| IBIS file stm32u595_599_5a5_5a9_ufbga132.ibs
[IBIS ver] 4.2
[File name] stm32u595_599_5a5_5a9_ufbga132.ibs
[File Rev] rev2.0
[Date]  11-09-2023
[Source] Data Created at STMicroelectronics
[Notes]  File originated from ELDO simulations.
[Disclaimer]  This information is for modeling purpose only and is
   not guaranteed. The information is subject to change without
   notice.
[Copyright] Copyright 2023 STMicroelectronics Inc.
|   Component stm32u595_599_5a5_5a9_ufbga132
[Component] stm32u595_599_5a5_5a9_ufbga132
[Manufacturer] STMicroelectronics
[Package]
| variable   typ   min   max
R_pkg  0  NA  NA
L_pkg  0  NA  NA
C_pkg  0  NA  NA
[Pin]   signal_name   model_name
A1  PE5  io8_100m_hslv_tamp_ft
A2  PE3  io8_100m_hslv_tamp_ft
A3  PE1  io8_100m_hslv_ft
A4  PB9  io8_100m_i2c_ft
A5  PB6  io8_100m_i2c_ft
A6  PG12  io8_100m_hslv_ft
A7  PD6  io8_166m_hslv_ft
A8  PD5  io8_100m_hslv_ft
A9  PD2  io8_100m_ft
A10  PC11  io8_100m_hslv_ft
A11  PA15  nc
A12  VDDUSB  power
B1  VBAT  power
B2  PE4  io8_100m_hslv_tamp_ft
B3  PE2  io8_100m_hslv_ft
B4  PG15  io8_100m_hslv_ft
B5  PH3-BOOT0  nc
B6  PB4  io8_100m_i2c_ft
B7  PG9  io8_100m_hslv_ft
B8  PD4  io8_100m_hslv_ft
B9  PD1  io8_100m_hslv_ft
B10  PC12  io8_166m_hslv_ft
B11  PC10  io8_100m_ft
B12  PA12  io8_100m_ft
C1  PC14-OSC32_IN  nc
C2  PE6  io8_100m_hslv_tamp_ft
C3  PC13  io8_100m_ft
C4  PE0  io8_100m_hslv_ft
C5  PB8  io8_100m_i2c_ft
C6  PB3  io8_100m_i2c_ft
C7  PG10  io8_100m_hslv_ft
C8  PD3  io8_166m_hslv_ft
C9  PD0  io8_100m_hslv_ft
C10  PA13  io8_100m_ft
C11  PA14  io8_100m_ft
C12  PA11  io8_100m_ft
D1  PC15-OSC32_OUT   nc
D2  PF0  io8_100m_hslv_ft
D3  PF3  io8_100m_hslv_ft
D4  VDD  power
D5  PB7  io8_spi_hslv_ft
D6  PB5  io8_166m_hslv_ft
D7  PD7  io8_100m_hslv_ft
D8  VDDIO2  power
D9  VDD  power
D10  PA9  io8_100m_usb_vbus_ft
D11  PA10  io8_100m_usb_id
D12  PA8  io8_166m_hslv_ft
E1  PF2  io8_100m_hslv_ft
E2  PF1  io8_100m_hslv_ft
E3  PF4  io8_spi_ft
E4  VSS  gnd
E9  VSS  gnd
E10  PC7  io8_100m_ft
E11  PC9  io8_100m_ft
E12  PC8  io8_100m_ft
F1  PH0-OSC_IN   nc
F2  PF5  io8_spi_ft
F3  PC2  io8_100m_hslv_ft
F4  PC3  io8_100m_hslv_ft
F6  VSS  gnd
F7  VDD  power
F9  PG6  io8_100m_hslv_ft
F10  PG7  io8_100m_hslv_ft
F11  PC6  io8_100m_ft
F12  PG8  io8_100m_i2c_ft
G1  PH1-OSC_OUT   nc
G2  NRST  nc
G3  PC1  io8_spi_hslv_ft
G4  PA1  io8_100m_hslv_tamp_ft
G6  VDD  power
G7  VSS  gnd
G9  PG4  io8_100m_hslv_ft
G10  PG2  io8_100m_hslv_ft
G11  PG3  io8_100m_hslv_ft
G12  PG5  io8_100m_hslv_ft
H1  VSSA_VREFM  nc
H2  PC0  io8_100m_hslv_ft
H3  OPAMP1_VINM  nc
H4  VSS  gnd
H9  VSS  gnd
H10  PD14  io8_100m_hslv_ft
H11  PD13  io8_100m_hslv_ft
H12  PD15  io8_100m_hslv_ft
J1  VREFP  nc
J2  PA0  io8_100m_hslv_tamp_ft
J3  PC5  io8_100m_tamp_ft
J4  VDD  power
J5  PF14  io8_100m_hslv_ft
J6  PE8  io8_100m_hslv_ft
J7  PE10  io8_166m_hslv_ft
J8  PE12  io8_100m_hslv_ft
J9  VDD  power
J10  PD9  io8_100m_hslv_ft
J11  PD11  io8_100m_hslv_ft
J12  PD12  io8_100m_hslv_ft
K1  VDDA  nc
K2  PA2  io8_100m_hslv_ft
K3  PA7  io8_100m_hslv_ft
K4  PB2  io8_100m_hslv_tamp_ft
K5  PF11  io8_166m_hslv_ft
K6  PG1  io8_100m_hslv_ft
K7  PE7  io8_100m_hslv_ft
K8  PE14  io8_100m_hslv_ft
K9  PB10  io8_spi_hslv_ft
K10  PB13  io8_100m_i2c_ft
K11  PB14  io8_100m_i2c_ft
K12  PB15  nc
L1  PA3  io8_166m_hslv_ft
L2  PA6  io8_100m_hslv_ft
L3  PA4  io8_100m_hslv_ft
L4  PB1  io8_100m_hslv_ft
L5  PF12  io8_100m_hslv_ft
L6  PF15  io8_100m_hslv_ft
L7  PE11  io8_100m_hslv_ft
L8  PE15  io8_100m_hslv_ft
L9  PB11  io8_100m_hslv_ft
L10  VCAP  nc
L11  PB12  io8_166m_hslv_ft
L12  PD8  io8_100m_hslv_ft
M1  PA5  io8_100m_ft
M2  OPAMP2_VINM  nc
M3  PC4  io8_100m_hslv_ft
M4  PB0  io8_100m_hslv_ft
M5  PF13  io8_100m_hslv_ft
M6  PG0  io8_100m_hslv_ft
M7  PE9  io8_166m_hslv_ft
M8  PE13  io8_100m_hslv_ft
M9  PG14  io8_100m_hslv_ft
M10  PG13  io8_100m_hslv_ft
M11  PG11  io8_100m_hslv_ft
M12  PD10  io8_100m_hslv_ft
[Package Model]   481-ufbga-7x7-132-ldo-220909
[Pin Mapping]   pulldown_ref   pullup_ref   | Comment
A1  gndio  vddiom
A2  gndio  vddiom
A3  gndio  vddiom
A4  gndio  vddiom
A5  gndio  vddiom
A6  gndio  vddiom  | Depending on IO usage
| A6  gndio  vddio2  | Depending on IO usage
A7  gndio  vddiom
A8  gndio  vddiom
A9  gndio  vddiom
A10  gndio  vddiom
A11  nc  nc
A12  nc  vddusb
B1  nc  vsw
B2  gndio  vddiom
B3  gndio  vddiom
B4  gndio  vddiom  | Depending on IO usage
| B4  gndio  vddio2  | Depending on IO usage
B5  nc  nc
B6  gndio  vddiom
B7  gndio  vddiom  | Depending on IO usage
| B7  gndio  vddio2  | Depending on IO usage
B8  gndio  vddiom
B9  gndio  vddiom
B10  gndio  vddiom
B11  gndio  vddiom
B12  gndio  vddiom  | Depending on IO usage
| B12  gndio  vddusb  | Depending on IO usage
C1  nc  nc
C2  gndio  vddiom
C3  gndio  vddiom  | Depending on IO usage
| C3  gndio  vsw  | Depending on IO usage
C4  gndio  vddiom
C5  gndio  vddiom
C6  gndio  vddiom
C7  gndio  vddiom  | Depending on IO usage
| C7  gndio  vddio2  | Depending on IO usage
C8  gndio  vddiom
C9  gndio  vddiom
C10  gndio  vddiom  | Depending on IO usage
| C10  gndio  vddusb  | Depending on IO usage
C11  gndio  vddiom
C12  gndio  vddiom  | Depending on IO usage
| C12  gndio  vddusb  | Depending on IO usage
D1  nc  nc
D2  gndio  vddiom
D3  gndio  vddiom
D4  nc  vddiom
D5  gndio  vddiom
D6  gndio  vddiom
D7  gndio  vddiom
D8  nc  vddio2
D9  nc  vddiom
D10  gndio  vddiom  | Depending on IO usage
| D10  gndio  vddusb  | Depending on IO usage
D11  gndio  vddiom  | Depending on IO usage
| D11  gndio  vddusb  | Depending on IO usage
D12  gndio  vddiom
E1  gndio  vddiom
E2  gndio  vddiom
E3  gndio  vddiom
E4  gndio  nc
E9  gndio  nc
E10  gndio  vddiom
E11  gndio  vddiom
E12  gndio  vddiom
F1  nc  nc
F2  gndio  vddiom
F3  gndio  vddiom
F4  gndio  vddiom
F6  gndio  nc
F7  nc  vddiom
F9  gndio  vddiom  | Depending on IO usage
| F9  gndio  vddio2  | Depending on IO usage
F10  gndio  vddiom  | Depending on IO usage
| F10  gndio  vddio2  | Depending on IO usage
F11  gndio  vddiom
F12  gndio  vddiom  | Depending on IO usage
| F12  gndio  vddio2  | Depending on IO usage
G1  nc  nc
G2  nc  nc
G3  gndio  vddiom
G4  gndio  vddiom
G6  nc  vddiom
G7  gndio  nc
G9  gndio  vddiom  | Depending on IO usage
| G9  gndio  vddio2  | Depending on IO usage
G10  gndio  vddiom  | Depending on IO usage
| G10  gndio  vddio2  | Depending on IO usage
G11  gndio  vddiom  | Depending on IO usage
| G11  gndio  vddio2  | Depending on IO usage
G12  gndio  vddiom  | Depending on IO usage
| G12  gndio  vddio2  | Depending on IO usage
H1  nc  nc
H2  gndio  vddiom
H3  nc  nc
H4  gndio  nc
H9  gndio  nc
H10  gndio  vddiom
H11  gndio  vddiom
H12  gndio  vddiom
J1  nc  nc
J2  gndio  vddiom
J3  gndio  vddiom
J4  nc  vddiom
J5  gndio  vddiom
J6  gndio  vddiom
J7  gndio  vddiom
J8  gndio  vddiom
J9  nc  vddiom
J10  gndio  vddiom
J11  gndio  vddiom
J12  gndio  vddiom
K1  nc  nc
K2  gndio  vddiom
K3  gndio  vddiom
K4  gndio  vddiom
K5  gndio  vddiom
K6  gndio  vddiom
K7  gndio  vddiom
K8  gndio  vddiom
K9  gndio  vddiom
K10  gndio  vddiom
K11  gndio  vddiom
K12  nc  nc
L1  gndio  vddiom
L2  gndio  vddiom
L3  gndio  vddiom
L4  gndio  vddiom
L5  gndio  vddiom
L6  gndio  vddiom
L7  gndio  vddiom
L8  gndio  vddiom
L9  gndio  vddiom
L10  nc  nc
L11  gndio  vddiom
L12  gndio  vddiom
M1  gndio  vddiom
M2  nc  nc
M3  gndio  vddiom
M4  gndio  vddiom
M5  gndio  vddiom
M6  gndio  vddiom
M7  gndio  vddiom
M8  gndio  vddiom
M9  gndio  vddiom  | Depending on IO usage
| M9  gndio  vddio2  | Depending on IO usage
M10  gndio  vddiom  | Depending on IO usage
| M10  gndio  vddio2  | Depending on IO usage
M11  gndio  vddiom  | Depending on IO usage
| M11  gndio  vddio2  | Depending on IO usage
M12  gndio  vddiom
[Model Selector] io8_100m_ft
io8_100m_ft_hs_1v2  "IO8_FT 100MHz high speed @ 1.2V"
io8_100m_ft_fs_1v2  "IO8_FT 100MHz fast speed @ 1.2V"
io8_100m_ft_fs_pd_1v2  "IO8_FT 100MHz fast speed @ 1.2V pulldown"
io8_100m_ft_ms_1v2  "IO8_FT 100MHz med speed @ 1.2V"
io8_100m_ft_ms_pd_1v2  "IO8_FT 100MHz med speed @ 1.2V pulldown"
io8_100m_ft_ls_1v2  "IO8_FT 100MHz low speed @ 1.2V"
io8_100m_ft_ls_pd_1v2  "IO8_FT 100MHz low speed @ 1.2V pulldown"
io8_100m_ft_hs_1v8  "IO8_FT 100MHz high speed @ 1.8V"
io8_100m_ft_hs_pd_1v8  "IO8_FT 100MHz high speed @ 1.8V pulldown"
io8_100m_ft_fs_1v8  "IO8_FT 100MHz fast speed @ 1.8V"
io8_100m_ft_fs_pd_1v8  "IO8_FT 100MHz fast speed @ 1.8V pulldown"
io8_100m_ft_ms_1v8  "IO8_FT 100MHz med speed @ 1.8V"
io8_100m_ft_ms_pd_1v8  "IO8_FT 100MHz med speed @ 1.8V pulldown"
io8_100m_ft_ls_1v8  "IO8_FT 100MHz low speed @ 1.8V"
io8_100m_ft_ls_pd_1v8  "IO8_FT 100MHz low speed @ 1.8V pulldown"
io8_100m_ft_hs_3v3  "IO8_FT 100MHz high speed @ 3.3V"
io8_100m_ft_hs_pd_3v3  "IO8_FT 100MHz high speed @ 3.3V pulldown"
io8_100m_ft_fs_3v3  "IO8_FT 100MHz fast speed @ 3.3V"
io8_100m_ft_fs_pd_3v3  "IO8_FT 100MHz fast speed @ 3.3V pulldown"
io8_100m_ft_ms_3v3  "IO8_FT 100MHz med speed @ 3.3V"
io8_100m_ft_ms_pd_3v3  "IO8_FT 100MHz med speed @ 3.3V pulldown"
io8_100m_ft_ls_3v3  "IO8_FT 100MHz low speed @ 3.3V"
io8_100m_ft_ls_pd_3v3  "IO8_FT 100MHz low speed @ 3.3V pulldown"
[Model Selector] io8_100m_hslv_ft
io8_100m_ft_hs_1v2  "IO8_FT 100MHz high speed @ 1.2V"
io8_100m_ft_hs_pu_1v2  "IO8_FT 100MHz high speed @ 1.2V pullup"
io8_100m_ft_hs_pd_1v2  "IO8_FT 100MHz high speed @ 1.2V pulldown"
io8_100m_ft_fs_1v2  "IO8_FT 100MHz fast speed @ 1.2V"
io8_100m_ft_fs_pu_1v2  "IO8_FT 100MHz fast speed @ 1.2V pullup"
io8_100m_ft_fs_pd_1v2  "IO8_FT 100MHz fast speed @ 1.2V pulldown"
io8_100m_ft_ms_1v2  "IO8_FT 100MHz med speed @ 1.2V"
io8_100m_ft_ms_pu_1v2  "IO8_FT 100MHz med speed @ 1.2V pullup"
io8_100m_ft_ms_pd_1v2  "IO8_FT 100MHz med speed @ 1.2V pulldown"
io8_100m_ft_ls_1v2  "IO8_FT 100MHz low speed @ 1.2V"
io8_100m_ft_ls_pu_1v2  "IO8_FT 100MHz low speed @ 1.2V pullup"
io8_100m_ft_ls_pd_1v2  "IO8_FT 100MHz low speed @ 1.2V pulldown"
io8_100m_ft_hs_1v8  "IO8_FT 100MHz high speed @ 1.8V"
io8_100m_ft_hs_pu_1v8  "IO8_FT 100MHz high speed @ 1.8V pullup"
io8_100m_ft_hs_pd_1v8  "IO8_FT 100MHz high speed @ 1.8V pulldown"
io8_100m_ft_fs_1v8  "IO8_FT 100MHz fast speed @ 1.8V"
io8_100m_ft_fs_pu_1v8  "IO8_FT 100MHz fast speed @ 1.8V pullup"
io8_100m_ft_fs_pd_1v8  "IO8_FT 100MHz fast speed @ 1.8V pulldown"
io8_100m_ft_ms_1v8  "IO8_FT 100MHz med speed @ 1.8V"
io8_100m_ft_ms_pu_1v8  "IO8_FT 100MHz med speed @ 1.8V pullup"
io8_100m_ft_ms_pd_1v8  "IO8_FT 100MHz med speed @ 1.8V pulldown"
io8_100m_ft_ls_1v8  "IO8_FT 100MHz low speed @ 1.8V"
io8_100m_ft_ls_pu_1v8  "IO8_FT 100MHz low speed @ 1.8V pullup"
io8_100m_ft_ls_pd_1v8  "IO8_FT 100MHz low speed @ 1.8V pulldown"
io8_100m_ft_hs_3v3  "IO8_FT 100MHz high speed @ 3.3V"
io8_100m_ft_hs_pu_3v3  "IO8_FT 100MHz high speed @ 3.3V pullup"
io8_100m_ft_hs_pd_3v3  "IO8_FT 100MHz high speed @ 3.3V pulldown"
io8_100m_ft_fs_3v3  "IO8_FT 100MHz fast speed @ 3.3V"
io8_100m_ft_fs_pu_3v3  "IO8_FT 100MHz fast speed @ 3.3V pullup"
io8_100m_ft_fs_pd_3v3  "IO8_FT 100MHz fast speed @ 3.3V pulldown"
io8_100m_ft_ms_3v3  "IO8_FT 100MHz med speed @ 3.3V"
io8_100m_ft_ms_pu_3v3  "IO8_FT 100MHz med speed @ 3.3V pullup"
io8_100m_ft_ms_pd_3v3  "IO8_FT 100MHz med speed @ 3.3V pulldown"
io8_100m_ft_ls_3v3  "IO8_FT 100MHz low speed @ 3.3V"
io8_100m_ft_ls_pu_3v3  "IO8_FT 100MHz low speed @ 3.3V pullup"
io8_100m_ft_ls_pd_3v3  "IO8_FT 100MHz low speed @ 3.3V pulldown"
io8_100m_hslv_ft_hs_1v2  "IO8_FT 100MHz HSLV high speed @ 1.2V"
io8_100m_hslv_ft_hs_pu_1v2  "IO8_FT 100MHz HSLV high speed @ 1.2V pullup"
io8_100m_hslv_ft_hs_pd_1v2  "IO8_FT 100MHz HSLV high speed @ 1.2V pulldown"
io8_100m_hslv_ft_fs_1v2  "IO8_FT 100MHz HSLV fast speed @ 1.2V"
io8_100m_hslv_ft_fs_pu_1v2  "IO8_FT 100MHz HSLV fast speed @ 1.2V pullup"
io8_100m_hslv_ft_fs_pd_1v2  "IO8_FT 100MHz HSLV fast speed @ 1.2V pulldown"
io8_100m_hslv_ft_ms_1v2  "IO8_FT 100MHz HSLV med speed @ 1.2V"
io8_100m_hslv_ft_ms_pu_1v2  "IO8_FT 100MHz HSLV med speed @ 1.2V pullup"
io8_100m_hslv_ft_ms_pd_1v2  "IO8_FT 100MHz HSLV med speed @ 1.2V pulldown"
io8_100m_hslv_ft_ls_1v2  "IO8_FT 100MHz HSLV low speed @ 1.2V"
io8_100m_hslv_ft_ls_pu_1v2  "IO8_FT 100MHz HSLV low speed @ 1.2V pullup"
io8_100m_hslv_ft_ls_pd_1v2  "IO8_FT 100MHz HSLV low speed @ 1.2V pulldown"
io8_100m_hslv_ft_hs_1v8  "IO8_FT 100MHz HSLV high speed @ 1.8V"
io8_100m_hslv_ft_hs_pu_1v8  "IO8_FT 100MHz HSLV high speed @ 1.8V pullup"
io8_100m_hslv_ft_hs_pd_1v8  "IO8_FT 100MHz HSLV high speed @ 1.8V pulldown"
io8_100m_hslv_ft_fs_1v8  "IO8_FT 100MHz HSLV fast speed @ 1.8V"
io8_100m_hslv_ft_fs_pu_1v8  "IO8_FT 100MHz HSLV fast speed @ 1.8V pullup"
io8_100m_hslv_ft_fs_pd_1v8  "IO8_FT 100MHz HSLV fast speed @ 1.8V pulldown"
io8_100m_hslv_ft_ms_1v8  "IO8_FT 100MHz HSLV med speed @ 1.8V"
io8_100m_hslv_ft_ms_pu_1v8  "IO8_FT 100MHz HSLV med speed @ 1.8V pullup"
io8_100m_hslv_ft_ms_pd_1v8  "IO8_FT 100MHz HSLV med speed @ 1.8V pulldown"
io8_100m_hslv_ft_ls_1v8  "IO8_FT 100MHz HSLV low speed @ 1.8V"
io8_100m_hslv_ft_ls_pu_1v8  "IO8_FT 100MHz HSLV low speed @ 1.8V pullup"
io8_100m_hslv_ft_ls_pd_1v8  "IO8_FT 100MHz HSLV low speed @ 1.8V pulldown"
io8_100m_hslv_ft_hs_2v5  "IO8_FT 100MHz HSLV high speed @ 2.5V"
io8_100m_hslv_ft_hs_pu_2v5  "IO8_FT 100MHz HSLV high speed @ 2.5V pullup"
io8_100m_hslv_ft_hs_pd_2v5  "IO8_FT 100MHz HSLV high speed @ 2.5V pulldown"
io8_100m_hslv_ft_fs_2v5  "IO8_FT 100MHz HSLV fast speed @ 2.5V"
io8_100m_hslv_ft_fs_pu_2v5  "IO8_FT 100MHz HSLV fast speed @ 2.5V pullup"
io8_100m_hslv_ft_fs_pd_2v5  "IO8_FT 100MHz HSLV fast speed @ 2.5V pulldown"
io8_100m_hslv_ft_ms_2v5  "IO8_FT 100MHz HSLV med speed @ 2.5V"
io8_100m_hslv_ft_ms_pu_2v5  "IO8_FT 100MHz HSLV med speed @ 2.5V pullup"
io8_100m_hslv_ft_ms_pd_2v5  "IO8_FT 100MHz HSLV med speed @ 2.5V pulldown"
io8_100m_hslv_ft_ls_2v5  "IO8_FT 100MHz HSLV low speed @ 2.5V"
io8_100m_hslv_ft_ls_pu_2v5  "IO8_FT 100MHz HSLV low speed @ 2.5V pullup"
io8_100m_hslv_ft_ls_pd_2v5  "IO8_FT 100MHz HSLV low speed @ 2.5V pulldown"
[Model Selector] io8_100m_hslv_tamp_ft
io8_100m_ft_hs_1v2  "IO8_FT 100MHz high speed @ 1.2V"
io8_100m_ft_hs_pu_1v2  "IO8_FT 100MHz high speed @ 1.2V pullup"
io8_100m_ft_hs_pd_1v2  "IO8_FT 100MHz high speed @ 1.2V pulldown"
io8_100m_ft_fs_1v2  "IO8_FT 100MHz fast speed @ 1.2V"
io8_100m_ft_fs_pu_1v2  "IO8_FT 100MHz fast speed @ 1.2V pullup"
io8_100m_ft_fs_pd_1v2  "IO8_FT 100MHz fast speed @ 1.2V pulldown"
io8_100m_ft_ms_1v2  "IO8_FT 100MHz med speed @ 1.2V"
io8_100m_ft_ms_pu_1v2  "IO8_FT 100MHz med speed @ 1.2V pullup"
io8_100m_ft_ms_pd_1v2  "IO8_FT 100MHz med speed @ 1.2V pulldown"
io8_100m_ft_ls_1v2  "IO8_FT 100MHz low speed @ 1.2V"
io8_100m_ft_ls_pu_1v2  "IO8_FT 100MHz low speed @ 1.2V pullup"
io8_100m_ft_ls_pd_1v2  "IO8_FT 100MHz low speed @ 1.2V pulldown"
io8_100m_ft_hs_1v8  "IO8_FT 100MHz high speed @ 1.8V"
io8_100m_ft_hs_pu_1v8  "IO8_FT 100MHz high speed @ 1.8V pullup"
io8_100m_ft_hs_pd_1v8  "IO8_FT 100MHz high speed @ 1.8V pulldown"
io8_100m_ft_fs_1v8  "IO8_FT 100MHz fast speed @ 1.8V"
io8_100m_ft_fs_pu_1v8  "IO8_FT 100MHz fast speed @ 1.8V pullup"
io8_100m_ft_fs_pd_1v8  "IO8_FT 100MHz fast speed @ 1.8V pulldown"
io8_100m_ft_ms_1v8  "IO8_FT 100MHz med speed @ 1.8V"
io8_100m_ft_ms_pu_1v8  "IO8_FT 100MHz med speed @ 1.8V pullup"
io8_100m_ft_ms_pd_1v8  "IO8_FT 100MHz med speed @ 1.8V pulldown"
io8_100m_ft_ls_1v8  "IO8_FT 100MHz low speed @ 1.8V"
io8_100m_ft_ls_pu_1v8  "IO8_FT 100MHz low speed @ 1.8V pullup"
io8_100m_ft_ls_pd_1v8  "IO8_FT 100MHz low speed @ 1.8V pulldown"
io8_100m_ft_hs_3v3  "IO8_FT 100MHz high speed @ 3.3V"
io8_100m_ft_hs_pu_3v3  "IO8_FT 100MHz high speed @ 3.3V pullup"
io8_100m_ft_hs_pd_3v3  "IO8_FT 100MHz high speed @ 3.3V pulldown"
io8_100m_ft_fs_3v3  "IO8_FT 100MHz fast speed @ 3.3V"
io8_100m_ft_fs_pu_3v3  "IO8_FT 100MHz fast speed @ 3.3V pullup"
io8_100m_ft_fs_pd_3v3  "IO8_FT 100MHz fast speed @ 3.3V pulldown"
io8_100m_ft_ms_3v3  "IO8_FT 100MHz med speed @ 3.3V"
io8_100m_ft_ms_pu_3v3  "IO8_FT 100MHz med speed @ 3.3V pullup"
io8_100m_ft_ms_pd_3v3  "IO8_FT 100MHz med speed @ 3.3V pulldown"
io8_100m_ft_ls_3v3  "IO8_FT 100MHz low speed @ 3.3V"
io8_100m_ft_ls_pu_3v3  "IO8_FT 100MHz low speed @ 3.3V pullup"
io8_100m_ft_ls_pd_3v3  "IO8_FT 100MHz low speed @ 3.3V pulldown"
io8_100m_hslv_ft_hs_1v2  "IO8_FT 100MHz HSLV high speed @ 1.2V"
io8_100m_hslv_ft_hs_pu_1v2  "IO8_FT 100MHz HSLV high speed @ 1.2V pullup"
io8_100m_hslv_ft_hs_pd_1v2  "IO8_FT 100MHz HSLV high speed @ 1.2V pulldown"
io8_100m_hslv_ft_fs_1v2  "IO8_FT 100MHz HSLV fast speed @ 1.2V"
io8_100m_hslv_ft_fs_pu_1v2  "IO8_FT 100MHz HSLV fast speed @ 1.2V pullup"
io8_100m_hslv_ft_fs_pd_1v2  "IO8_FT 100MHz HSLV fast speed @ 1.2V pulldown"
io8_100m_hslv_ft_ms_1v2  "IO8_FT 100MHz HSLV med speed @ 1.2V"
io8_100m_hslv_ft_ms_pu_1v2  "IO8_FT 100MHz HSLV med speed @ 1.2V pullup"
io8_100m_hslv_ft_ms_pd_1v2  "IO8_FT 100MHz HSLV med speed @ 1.2V pulldown"
io8_100m_hslv_ft_ls_1v2  "IO8_FT 100MHz HSLV low speed @ 1.2V"
io8_100m_hslv_ft_ls_pu_1v2  "IO8_FT 100MHz HSLV low speed @ 1.2V pullup"
io8_100m_hslv_ft_ls_pd_1v2  "IO8_FT 100MHz HSLV low speed @ 1.2V pulldown"
io8_100m_hslv_ft_hs_1v8  "IO8_FT 100MHz HSLV high speed @ 1.8V"
io8_100m_hslv_ft_hs_pu_1v8  "IO8_FT 100MHz HSLV high speed @ 1.8V pullup"
io8_100m_hslv_ft_hs_pd_1v8  "IO8_FT 100MHz HSLV high speed @ 1.8V pulldown"
io8_100m_hslv_ft_fs_1v8  "IO8_FT 100MHz HSLV fast speed @ 1.8V"
io8_100m_hslv_ft_fs_pu_1v8  "IO8_FT 100MHz HSLV fast speed @ 1.8V pullup"
io8_100m_hslv_ft_fs_pd_1v8  "IO8_FT 100MHz HSLV fast speed @ 1.8V pulldown"
io8_100m_hslv_ft_ms_1v8  "IO8_FT 100MHz HSLV med speed @ 1.8V"
io8_100m_hslv_ft_ms_pu_1v8  "IO8_FT 100MHz HSLV med speed @ 1.8V pullup"
io8_100m_hslv_ft_ms_pd_1v8  "IO8_FT 100MHz HSLV med speed @ 1.8V pulldown"
io8_100m_hslv_ft_ls_1v8  "IO8_FT 100MHz HSLV low speed @ 1.8V"
io8_100m_hslv_ft_ls_pu_1v8  "IO8_FT 100MHz HSLV low speed @ 1.8V pullup"
io8_100m_hslv_ft_ls_pd_1v8  "IO8_FT 100MHz HSLV low speed @ 1.8V pulldown"
io8_100m_hslv_ft_hs_2v5  "IO8_FT 100MHz HSLV high speed @ 2.5V"
io8_100m_hslv_ft_hs_pu_2v5  "IO8_FT 100MHz HSLV high speed @ 2.5V pullup"
io8_100m_hslv_ft_hs_pd_2v5  "IO8_FT 100MHz HSLV high speed @ 2.5V pulldown"
io8_100m_hslv_ft_fs_2v5  "IO8_FT 100MHz HSLV fast speed @ 2.5V"
io8_100m_hslv_ft_fs_pu_2v5  "IO8_FT 100MHz HSLV fast speed @ 2.5V pullup"
io8_100m_hslv_ft_fs_pd_2v5  "IO8_FT 100MHz HSLV fast speed @ 2.5V pulldown"
io8_100m_hslv_ft_ms_2v5  "IO8_FT 100MHz HSLV med speed @ 2.5V"
io8_100m_hslv_ft_ms_pu_2v5  "IO8_FT 100MHz HSLV med speed @ 2.5V pullup"
io8_100m_hslv_ft_ms_pd_2v5  "IO8_FT 100MHz HSLV med speed @ 2.5V pulldown"
io8_100m_hslv_ft_ls_2v5  "IO8_FT 100MHz HSLV low speed @ 2.5V"
io8_100m_hslv_ft_ls_pu_2v5  "IO8_FT 100MHz HSLV low speed @ 2.5V pullup"
io8_100m_hslv_ft_ls_pd_2v5  "IO8_FT 100MHz HSLV low speed @ 2.5V pulldown"
io8_ft_v33_hs_1v2  "IO8_FT_V33 high speed @ 1.2V"
io8_ft_v33_hs_pu_1v2  "IO8_FT_V33 high speed @ 1.2V pullup"
io8_ft_v33_hs_pd_1v2  "IO8_FT_V33 high speed @ 1.2V pulldown"
io8_ft_v33_fs_1v2  "IO8_FT_V33 fast speed @ 1.2V"
io8_ft_v33_fs_pu_1v2  "IO8_FT_V33 fast speed @ 1.2V pullup"
io8_ft_v33_fs_pd_1v2  "IO8_FT_V33 fast speed @ 1.2V pulldown"
io8_ft_v33_ms_1v2  "IO8_FT_V33 med speed @ 1.2V"
io8_ft_v33_ms_pu_1v2  "IO8_FT_V33 med speed @ 1.2V pullup"
io8_ft_v33_ms_pd_1v2  "IO8_FT_V33 med speed @ 1.2V pulldown"
io8_ft_v33_ls_1v2  "IO8_FT_V33 low speed @ 1.2V"
io8_ft_v33_ls_pu_1v2  "IO8_FT_V33 low speed @ 1.2V pullup"
io8_ft_v33_ls_pd_1v2  "IO8_FT_V33 low speed @ 1.2V pulldown"
io8_ft_v33_hs_1v8  "IO8_FT_V33 high speed @ 1.8V"
io8_ft_v33_hs_pu_1v8  "IO8_FT_V33 high speed @ 1.8V pullup"
io8_ft_v33_hs_pd_1v8  "IO8_FT_V33 high speed @ 1.8V pulldown"
io8_ft_v33_fs_1v8  "IO8_FT_V33 fast speed @ 1.8V"
io8_ft_v33_fs_pu_1v8  "IO8_FT_V33 fast speed @ 1.8V pullup"
io8_ft_v33_fs_pd_1v8  "IO8_FT_V33 fast speed @ 1.8V pulldown"
io8_ft_v33_ms_1v8  "IO8_FT_V33 med speed @ 1.8V"
io8_ft_v33_ms_pu_1v8  "IO8_FT_V33 med speed @ 1.8V pullup"
io8_ft_v33_ms_pd_1v8  "IO8_FT_V33 med speed @ 1.8V pulldown"
io8_ft_v33_ls_1v8  "IO8_FT_V33 low speed @ 1.8V"
io8_ft_v33_ls_pu_1v8  "IO8_FT_V33 low speed @ 1.8V pullup"
io8_ft_v33_ls_pd_1v8  "IO8_FT_V33 low speed @ 1.8V pulldown"
io8_ft_v33_hs_3v3  "IO8_FT_V33 high speed @ 3.3V"
io8_ft_v33_hs_pu_3v3  "IO8_FT_V33 high speed @ 3.3V pullup"
io8_ft_v33_hs_pd_3v3  "IO8_FT_V33 high speed @ 3.3V pulldown"
io8_ft_v33_fs_3v3  "IO8_FT_V33 fast speed @ 3.3V"
io8_ft_v33_fs_pu_3v3  "IO8_FT_V33 fast speed @ 3.3V pullup"
io8_ft_v33_fs_pd_3v3  "IO8_FT_V33 fast speed @ 3.3V pulldown"
io8_ft_v33_ms_3v3  "IO8_FT_V33 med speed @ 3.3V"
io8_ft_v33_ms_pu_3v3  "IO8_FT_V33 med speed @ 3.3V pullup"
io8_ft_v33_ms_pd_3v3  "IO8_FT_V33 med speed @ 3.3V pulldown"
io8_ft_v33_ls_3v3  "IO8_FT_V33 low speed @ 3.3V"
io8_ft_v33_ls_pu_3v3  "IO8_FT_V33 low speed @ 3.3V pullup"
io8_ft_v33_ls_pd_3v3  "IO8_FT_V33 low speed @ 3.3V pulldown"
[Model Selector] io8_100m_i2c_ft
io8_100m_ft_hs_1v2  "IO8_FT 100MHz high speed @ 1.2V"
io8_100m_ft_hs_pu_1v2  "IO8_FT 100MHz high speed @ 1.2V pullup"
io8_100m_ft_hs_pd_1v2  "IO8_FT 100MHz high speed @ 1.2V pulldown"
io8_100m_ft_fs_1v2  "IO8_FT 100MHz fast speed @ 1.2V"
io8_100m_ft_fs_pu_1v2  "IO8_FT 100MHz fast speed @ 1.2V pullup"
io8_100m_ft_fs_pd_1v2  "IO8_FT 100MHz fast speed @ 1.2V pulldown"
io8_100m_ft_ms_1v2  "IO8_FT 100MHz med speed @ 1.2V"
io8_100m_ft_ms_pu_1v2  "IO8_FT 100MHz med speed @ 1.2V pullup"
io8_100m_ft_ms_pd_1v2  "IO8_FT 100MHz med speed @ 1.2V pulldown"
io8_100m_ft_ls_1v2  "IO8_FT 100MHz low speed @ 1.2V"
io8_100m_ft_ls_pu_1v2  "IO8_FT 100MHz low speed @ 1.2V pullup"
io8_100m_ft_ls_pd_1v2  "IO8_FT 100MHz low speed @ 1.2V pulldown"
io8_100m_ft_hs_1v8  "IO8_FT 100MHz high speed @ 1.8V"
io8_100m_ft_hs_pu_1v8  "IO8_FT 100MHz high speed @ 1.8V pullup"
io8_100m_ft_hs_pd_1v8  "IO8_FT 100MHz high speed @ 1.8V pulldown"
io8_100m_ft_fs_1v8  "IO8_FT 100MHz fast speed @ 1.8V"
io8_100m_ft_fs_pu_1v8  "IO8_FT 100MHz fast speed @ 1.8V pullup"
io8_100m_ft_fs_pd_1v8  "IO8_FT 100MHz fast speed @ 1.8V pulldown"
io8_100m_ft_ms_1v8  "IO8_FT 100MHz med speed @ 1.8V"
io8_100m_ft_ms_pu_1v8  "IO8_FT 100MHz med speed @ 1.8V pullup"
io8_100m_ft_ms_pd_1v8  "IO8_FT 100MHz med speed @ 1.8V pulldown"
io8_100m_ft_ls_1v8  "IO8_FT 100MHz low speed @ 1.8V"
io8_100m_ft_ls_pu_1v8  "IO8_FT 100MHz low speed @ 1.8V pullup"
io8_100m_ft_ls_pd_1v8  "IO8_FT 100MHz low speed @ 1.8V pulldown"
io8_100m_ft_hs_3v3  "IO8_FT 100MHz high speed @ 3.3V"
io8_100m_ft_hs_pu_3v3  "IO8_FT 100MHz high speed @ 3.3V pullup"
io8_100m_ft_hs_pd_3v3  "IO8_FT 100MHz high speed @ 3.3V pulldown"
io8_100m_ft_fs_3v3  "IO8_FT 100MHz fast speed @ 3.3V"
io8_100m_ft_fs_pu_3v3  "IO8_FT 100MHz fast speed @ 3.3V pullup"
io8_100m_ft_fs_pd_3v3  "IO8_FT 100MHz fast speed @ 3.3V pulldown"
io8_100m_ft_ms_3v3  "IO8_FT 100MHz med speed @ 3.3V"
io8_100m_ft_ms_pu_3v3  "IO8_FT 100MHz med speed @ 3.3V pullup"
io8_100m_ft_ms_pd_3v3  "IO8_FT 100MHz med speed @ 3.3V pulldown"
io8_100m_ft_ls_3v3  "IO8_FT 100MHz low speed @ 3.3V"
io8_100m_ft_ls_pu_3v3  "IO8_FT 100MHz low speed @ 3.3V pullup"
io8_100m_ft_ls_pd_3v3  "IO8_FT 100MHz low speed @ 3.3V pulldown"
io8_100m_i2c_ft_1v2  "IO8_FT 100MHz I2C @ 1.2V"
io8_100m_i2c_ft_pu_1v2  "IO8_FT 100MHz I2C @ 1.2V pullup"
io8_100m_i2c_ft_pd_1v2  "IO8_FT 100MHz I2C @ 1.2V pulldown"
io8_100m_i2c_ft_1v8  "IO8_FT 100MHz I2C @ 1.8V"
io8_100m_i2c_ft_pu_1v8  "IO8_FT 100MHz I2C @ 1.8V pullup"
io8_100m_i2c_ft_pd_1v8  "IO8_FT 100MHz I2C @ 1,8V pulldown"
io8_100m_i2c_ft_3v3  "IO8_FT 100MHz I2C @ 3.3V"
io8_100m_i2c_ft_pu_3v3  "IO8_FT 100MHz I2C HSLV @ 3.3V pullup"
io8_100m_i2c_ft_pd_3v3  "IO8_FT 100MHz I2C @ 3.3V pulldown"
[Model Selector] io8_100m_tamp_ft
io8_100m_ft_hs_1v2  "IO8_FT 100MHz high speed @ 1.2V"
io8_100m_ft_hs_pu_1v2  "IO8_FT 100MHz high speed @ 1.2V pullup"
io8_100m_ft_hs_pd_1v2  "IO8_FT 100MHz high speed @ 1.2V pulldown"
io8_100m_ft_fs_1v2  "IO8_FT 100MHz fast speed @ 1.2V"
io8_100m_ft_fs_pu_1v2  "IO8_FT 100MHz fast speed @ 1.2V pullup"
io8_100m_ft_fs_pd_1v2  "IO8_FT 100MHz fast speed @ 1.2V pulldown"
io8_100m_ft_ms_1v2  "IO8_FT 100MHz med speed @ 1.2V"
io8_100m_ft_ms_pu_1v2  "IO8_FT 100MHz med speed @ 1.2V pullup"
io8_100m_ft_ms_pd_1v2  "IO8_FT 100MHz med speed @ 1.2V pulldown"
io8_100m_ft_ls_1v2  "IO8_FT 100MHz low speed @ 1.2V"
io8_100m_ft_ls_pu_1v2  "IO8_FT 100MHz low speed @ 1.2V pullup"
io8_100m_ft_ls_pd_1v2  "IO8_FT 100MHz low speed @ 1.2V pulldown"
io8_100m_ft_hs_1v8  "IO8_FT 100MHz high speed @ 1.8V"
io8_100m_ft_hs_pu_1v8  "IO8_FT 100MHz high speed @ 1.8V pullup"
io8_100m_ft_hs_pd_1v8  "IO8_FT 100MHz high speed @ 1.8V pulldown"
io8_100m_ft_fs_1v8  "IO8_FT 100MHz fast speed @ 1.8V"
io8_100m_ft_fs_pu_1v8  "IO8_FT 100MHz fast speed @ 1.8V pullup"
io8_100m_ft_fs_pd_1v8  "IO8_FT 100MHz fast speed @ 1.8V pulldown"
io8_100m_ft_ms_1v8  "IO8_FT 100MHz med speed @ 1.8V"
io8_100m_ft_ms_pu_1v8  "IO8_FT 100MHz med speed @ 1.8V pullup"
io8_100m_ft_ms_pd_1v8  "IO8_FT 100MHz med speed @ 1.8V pulldown"
io8_100m_ft_ls_1v8  "IO8_FT 100MHz low speed @ 1.8V"
io8_100m_ft_ls_pu_1v8  "IO8_FT 100MHz low speed @ 1.8V pullup"
io8_100m_ft_ls_pd_1v8  "IO8_FT 100MHz low speed @ 1.8V pulldown"
io8_100m_ft_hs_3v3  "IO8_FT 100MHz high speed @ 3.3V"
io8_100m_ft_hs_pu_3v3  "IO8_FT 100MHz high speed @ 3.3V pullup"
io8_100m_ft_hs_pd_3v3  "IO8_FT 100MHz high speed @ 3.3V pulldown"
io8_100m_ft_fs_3v3  "IO8_FT 100MHz fast speed @ 3.3V"
io8_100m_ft_fs_pu_3v3  "IO8_FT 100MHz fast speed @ 3.3V pullup"
io8_100m_ft_fs_pd_3v3  "IO8_FT 100MHz fast speed @ 3.3V pulldown"
io8_100m_ft_ms_3v3  "IO8_FT 100MHz med speed @ 3.3V"
io8_100m_ft_ms_pu_3v3  "IO8_FT 100MHz med speed @ 3.3V pullup"
io8_100m_ft_ms_pd_3v3  "IO8_FT 100MHz med speed @ 3.3V pulldown"
io8_100m_ft_ls_3v3  "IO8_FT 100MHz low speed @ 3.3V"
io8_100m_ft_ls_pu_3v3  "IO8_FT 100MHz low speed @ 3.3V pullup"
io8_100m_ft_ls_pd_3v3  "IO8_FT 100MHz low speed @ 3.3V pulldown"
io8_ft_v33_hs_1v2  "IO8_FT_V33 high speed @ 1.2V"
io8_ft_v33_hs_pu_1v2  "IO8_FT_V33 high speed @ 1.2V pullup"
io8_ft_v33_hs_pd_1v2  "IO8_FT_V33 high speed @ 1.2V pulldown"
io8_ft_v33_fs_1v2  "IO8_FT_V33 fast speed @ 1.2V"
io8_ft_v33_fs_pu_1v2  "IO8_FT_V33 fast speed @ 1.2V pullup"
io8_ft_v33_fs_pd_1v2  "IO8_FT_V33 fast speed @ 1.2V pulldown"
io8_ft_v33_ms_1v2  "IO8_FT_V33 med speed @ 1.2V"
io8_ft_v33_ms_pu_1v2  "IO8_FT_V33 med speed @ 1.2V pullup"
io8_ft_v33_ms_pd_1v2  "IO8_FT_V33 med speed @ 1.2V pulldown"
io8_ft_v33_ls_1v2  "IO8_FT_V33 low speed @ 1.2V"
io8_ft_v33_ls_pu_1v2  "IO8_FT_V33 low speed @ 1.2V pullup"
io8_ft_v33_ls_pd_1v2  "IO8_FT_V33 low speed @ 1.2V pulldown"
io8_ft_v33_hs_1v8  "IO8_FT_V33 high speed @ 1.8V"
io8_ft_v33_hs_pu_1v8  "IO8_FT_V33 high speed @ 1.8V pullup"
io8_ft_v33_hs_pd_1v8  "IO8_FT_V33 high speed @ 1.8V pulldown"
io8_ft_v33_fs_1v8  "IO8_FT_V33 fast speed @ 1.8V"
io8_ft_v33_fs_pu_1v8  "IO8_FT_V33 fast speed @ 1.8V pullup"
io8_ft_v33_fs_pd_1v8  "IO8_FT_V33 fast speed @ 1.8V pulldown"
io8_ft_v33_ms_1v8  "IO8_FT_V33 med speed @ 1.8V"
io8_ft_v33_ms_pu_1v8  "IO8_FT_V33 med speed @ 1.8V pullup"
io8_ft_v33_ms_pd_1v8  "IO8_FT_V33 med speed @ 1.8V pulldown"
io8_ft_v33_ls_1v8  "IO8_FT_V33 low speed @ 1.8V"
io8_ft_v33_ls_pu_1v8  "IO8_FT_V33 low speed @ 1.8V pullup"
io8_ft_v33_ls_pd_1v8  "IO8_FT_V33 low speed @ 1.8V pulldown"
io8_ft_v33_hs_3v3  "IO8_FT_V33 high speed @ 3.3V"
io8_ft_v33_hs_pu_3v3  "IO8_FT_V33 high speed @ 3.3V pullup"
io8_ft_v33_hs_pd_3v3  "IO8_FT_V33 high speed @ 3.3V pulldown"
io8_ft_v33_fs_3v3  "IO8_FT_V33 fast speed @ 3.3V"
io8_ft_v33_fs_pu_3v3  "IO8_FT_V33 fast speed @ 3.3V pullup"
io8_ft_v33_fs_pd_3v3  "IO8_FT_V33 fast speed @ 3.3V pulldown"
io8_ft_v33_ms_3v3  "IO8_FT_V33 med speed @ 3.3V"
io8_ft_v33_ms_pu_3v3  "IO8_FT_V33 med speed @ 3.3V pullup"
io8_ft_v33_ms_pd_3v3  "IO8_FT_V33 med speed @ 3.3V pulldown"
io8_ft_v33_ls_3v3  "IO8_FT_V33 low speed @ 3.3V"
io8_ft_v33_ls_pu_3v3  "IO8_FT_V33 low speed @ 3.3V pullup"
io8_ft_v33_ls_pd_3v3  "IO8_FT_V33 low speed @ 3.3V pulldown"
[Model Selector] io8_100m_usb_id
io8_100m_ft_hs_1v2  "IO8_FT 100MHz high speed @ 1.2V"
io8_100m_ft_hs_pu_1v2  "IO8_FT 100MHz high speed @ 1.2V pullup"
io8_100m_ft_hs_pd_1v2  "IO8_FT 100MHz high speed @ 1.2V pulldown"
io8_100m_ft_fs_1v2  "IO8_FT 100MHz fast speed @ 1.2V"
io8_100m_ft_fs_pu_1v2  "IO8_FT 100MHz fast speed @ 1.2V pullup"
io8_100m_ft_fs_pd_1v2  "IO8_FT 100MHz fast speed @ 1.2V pulldown"
io8_100m_ft_ms_1v2  "IO8_FT 100MHz med speed @ 1.2V"
io8_100m_ft_ms_pu_1v2  "IO8_FT 100MHz med speed @ 1.2V pullup"
io8_100m_ft_ms_pd_1v2  "IO8_FT 100MHz med speed @ 1.2V pulldown"
io8_100m_ft_ls_1v2  "IO8_FT 100MHz low speed @ 1.2V"
io8_100m_ft_ls_pu_1v2  "IO8_FT 100MHz low speed @ 1.2V pullup"
io8_100m_ft_ls_pd_1v2  "IO8_FT 100MHz low speed @ 1.2V pulldown"
io8_100m_ft_hs_1v8  "IO8_FT 100MHz high speed @ 1.8V"
io8_100m_ft_hs_pu_1v8  "IO8_FT 100MHz high speed @ 1.8V pullup"
io8_100m_ft_hs_pd_1v8  "IO8_FT 100MHz high speed @ 1.8V pulldown"
io8_100m_ft_fs_1v8  "IO8_FT 100MHz fast speed @ 1.8V"
io8_100m_ft_fs_pu_1v8  "IO8_FT 100MHz fast speed @ 1.8V pullup"
io8_100m_ft_fs_pd_1v8  "IO8_FT 100MHz fast speed @ 1.8V pulldown"
io8_100m_ft_ms_1v8  "IO8_FT 100MHz med speed @ 1.8V"
io8_100m_ft_ms_pu_1v8  "IO8_FT 100MHz med speed @ 1.8V pullup"
io8_100m_ft_ms_pd_1v8  "IO8_FT 100MHz med speed @ 1.8V pulldown"
io8_100m_ft_ls_1v8  "IO8_FT 100MHz low speed @ 1.8V"
io8_100m_ft_ls_pu_1v8  "IO8_FT 100MHz low speed @ 1.8V pullup"
io8_100m_ft_ls_pd_1v8  "IO8_FT 100MHz low speed @ 1.8V pulldown"
io8_100m_ft_hs_3v3  "IO8_FT 100MHz high speed @ 3.3V"
io8_100m_ft_hs_pu_3v3  "IO8_FT 100MHz high speed @ 3.3V pullup"
io8_100m_ft_hs_pd_3v3  "IO8_FT 100MHz high speed @ 3.3V pulldown"
io8_100m_ft_fs_3v3  "IO8_FT 100MHz fast speed @ 3.3V"
io8_100m_ft_fs_pu_3v3  "IO8_FT 100MHz fast speed @ 3.3V pullup"
io8_100m_ft_fs_pd_3v3  "IO8_FT 100MHz fast speed @ 3.3V pulldown"
io8_100m_ft_ms_3v3  "IO8_FT 100MHz med speed @ 3.3V"
io8_100m_ft_ms_pu_3v3  "IO8_FT 100MHz med speed @ 3.3V pullup"
io8_100m_ft_ms_pd_3v3  "IO8_FT 100MHz med speed @ 3.3V pulldown"
io8_100m_ft_ls_3v3  "IO8_FT 100MHz low speed @ 3.3V"
io8_100m_ft_ls_pu_3v3  "IO8_FT 100MHz low speed @ 3.3V pullup"
io8_100m_ft_ls_pd_3v3  "IO8_FT 100MHz low speed @ 3.3V pulldown"
io8usb_id_nopu  "IOUSB ID @ 3.3V"
io8usb_id_pu  "IOUSB ID @ 3.3V pullup"
[Model Selector] io8_100m_usb_vbus_ft
io8_100m_ft_hs_1v2  "IO8_FT 100MHz high speed @ 1.2V"
io8_100m_ft_hs_pu_1v2  "IO8_FT 100MHz high speed @ 1.2V pullup"
io8_100m_ft_hs_pd_1v2  "IO8_FT 100MHz high speed @ 1.2V pulldown"
io8_100m_ft_fs_1v2  "IO8_FT 100MHz fast speed @ 1.2V"
io8_100m_ft_fs_pu_1v2  "IO8_FT 100MHz fast speed @ 1.2V pullup"
io8_100m_ft_fs_pd_1v2  "IO8_FT 100MHz fast speed @ 1.2V pulldown"
io8_100m_ft_ms_1v2  "IO8_FT 100MHz med speed @ 1.2V"
io8_100m_ft_ms_pu_1v2  "IO8_FT 100MHz med speed @ 1.2V pullup"
io8_100m_ft_ms_pd_1v2  "IO8_FT 100MHz med speed @ 1.2V pulldown"
io8_100m_ft_ls_1v2  "IO8_FT 100MHz low speed @ 1.2V"
io8_100m_ft_ls_pu_1v2  "IO8_FT 100MHz low speed @ 1.2V pullup"
io8_100m_ft_ls_pd_1v2  "IO8_FT 100MHz low speed @ 1.2V pulldown"
io8_100m_ft_hs_1v8  "IO8_FT 100MHz high speed @ 1.8V"
io8_100m_ft_hs_pu_1v8  "IO8_FT 100MHz high speed @ 1.8V pullup"
io8_100m_ft_hs_pd_1v8  "IO8_FT 100MHz high speed @ 1.8V pulldown"
io8_100m_ft_fs_1v8  "IO8_FT 100MHz fast speed @ 1.8V"
io8_100m_ft_fs_pu_1v8  "IO8_FT 100MHz fast speed @ 1.8V pullup"
io8_100m_ft_fs_pd_1v8  "IO8_FT 100MHz fast speed @ 1.8V pulldown"
io8_100m_ft_ms_1v8  "IO8_FT 100MHz med speed @ 1.8V"
io8_100m_ft_ms_pu_1v8  "IO8_FT 100MHz med speed @ 1.8V pullup"
io8_100m_ft_ms_pd_1v8  "IO8_FT 100MHz med speed @ 1.8V pulldown"
io8_100m_ft_ls_1v8  "IO8_FT 100MHz low speed @ 1.8V"
io8_100m_ft_ls_pu_1v8  "IO8_FT 100MHz low speed @ 1.8V pullup"
io8_100m_ft_ls_pd_1v8  "IO8_FT 100MHz low speed @ 1.8V pulldown"
io8_100m_ft_hs_3v3  "IO8_FT 100MHz high speed @ 3.3V"
io8_100m_ft_hs_pu_3v3  "IO8_FT 100MHz high speed @ 3.3V pullup"
io8_100m_ft_hs_pd_3v3  "IO8_FT 100MHz high speed @ 3.3V pulldown"
io8_100m_ft_fs_3v3  "IO8_FT 100MHz fast speed @ 3.3V"
io8_100m_ft_fs_pu_3v3  "IO8_FT 100MHz fast speed @ 3.3V pullup"
io8_100m_ft_fs_pd_3v3  "IO8_FT 100MHz fast speed @ 3.3V pulldown"
io8_100m_ft_ms_3v3  "IO8_FT 100MHz med speed @ 3.3V"
io8_100m_ft_ms_pu_3v3  "IO8_FT 100MHz med speed @ 3.3V pullup"
io8_100m_ft_ms_pd_3v3  "IO8_FT 100MHz med speed @ 3.3V pulldown"
io8_100m_ft_ls_3v3  "IO8_FT 100MHz low speed @ 3.3V"
io8_100m_ft_ls_pu_3v3  "IO8_FT 100MHz low speed @ 3.3V pullup"
io8_100m_ft_ls_pd_3v3  "IO8_FT 100MHz low speed @ 3.3V pulldown"
io8usb_adp "IOUSB ADP @ 3.3V"
io8usb_vbus "IOUSB VBUS @ 3.3V"
[Model Selector] io8_166m_hslv_ft
io8_166m_ft_hs_1v2  "IO8_FT 166MHz high speed @ 1.2V"
io8_166m_ft_hs_pu_1v2  "IO8_FT 166MHz high speed @ 1.2V pullup"
io8_166m_ft_hs_pd_1v2  "IO8_FT 166MHz high speed @ 1.2V pulldown"
io8_166m_ft_fs_1v2  "IO8_FT 166MHz fast speed @ 1.2V"
io8_166m_ft_fs_pu_1v2  "IO8_FT 166MHz fast speed @ 1.2V pullup"
io8_166m_ft_fs_pd_1v2  "IO8_FT 166MHz fast speed @ 1.2V pulldown"
io8_166m_ft_ms_1v2  "IO8_FT 166MHz med speed @ 1.2V"
io8_166m_ft_ms_pu_1v2  "IO8_FT 166MHz med speed @ 1.2V pullup"
io8_166m_ft_ms_pd_1v2  "IO8_FT 166MHz med speed @ 1.2V pulldown"
io8_166m_ft_ls_1v2  "IO8_FT 166MHz low speed @ 1.2V"
io8_166m_ft_ls_pu_1v2  "IO8_FT 166MHz low speed @ 1.2V pullup"
io8_166m_ft_ls_pd_1v2  "IO8_FT 166MHz low speed @ 1.2V pulldown"
io8_166m_ft_hs_1v8  "IO8_FT 166MHz high speed @ 1.8V"
io8_166m_ft_hs_pu_1v8  "IO8_FT 166MHz high speed @ 1.8V pullup"
io8_166m_ft_hs_pd_1v8  "IO8_FT 166MHz high speed @ 1.8V pulldown"
io8_166m_ft_fs_1v8  "IO8_FT 166MHz fast speed @ 1.8V"
io8_166m_ft_fs_pu_1v8  "IO8_FT 166MHz fast speed @ 1.8V pullup"
io8_166m_ft_fs_pd_1v8  "IO8_FT 166MHz fast speed @ 1.8V pulldown"
io8_166m_ft_ms_1v8  "IO8_FT 166MHz med speed @ 1.8V"
io8_166m_ft_ms_pu_1v8  "IO8_FT 166MHz med speed @ 1.8V pullup"
io8_166m_ft_ms_pd_1v8  "IO8_FT 166MHz med speed @ 1.8V pulldown"
io8_166m_ft_ls_1v8  "IO8_FT 166MHz low speed @ 1.8V"
io8_166m_ft_ls_pu_1v8  "IO8_FT 166MHz low speed @ 1.8V pullup"
io8_166m_ft_ls_pd_1v8  "IO8_FT 166MHz low speed @ 1.8V pulldown"
io8_166m_ft_hs_3v3  "IO8_FT 166MHz high speed @ 3.3V"
io8_166m_ft_hs_pu_3v3  "IO8_FT 166MHz high speed @ 3.3V pullup"
io8_166m_ft_hs_pd_3v3  "IO8_FT 166MHz high speed @ 3.3V pulldown"
io8_166m_ft_fs_3v3  "IO8_FT 166MHz fast speed @ 3.3V"
io8_166m_ft_fs_pu_3v3  "IO8_FT 166MHz fast speed @ 3.3V pullup"
io8_166m_ft_fs_pd_3v3  "IO8_FT 166MHz fast speed @ 3.3V pulldown"
io8_166m_ft_ms_3v3  "IO8_FT 166MHz med speed @ 3.3V"
io8_166m_ft_ms_pu_3v3  "IO8_FT 166MHz med speed @ 3.3V pullup"
io8_166m_ft_ms_pd_3v3  "IO8_FT 166MHz med speed @ 3.3V pulldown"
io8_166m_ft_ls_3v3  "IO8_FT 166MHz low speed @ 3.3V"
io8_166m_ft_ls_pu_3v3  "IO8_FT 166MHz low speed @ 3.3V pullup"
io8_166m_ft_ls_pd_3v3  "IO8_FT 166MHz low speed @ 3.3V pulldown"
io8_166m_hslv_ft_hs_1v2  "IO8_FT 166MHz HSLV high speed @ 1.2V"
io8_166m_hslv_ft_hs_pu_1v2  "IO8_FT 166MHz HSLV high speed @ 1.2V pullup"
io8_166m_hslv_ft_hs_pd_1v2  "IO8_FT 166MHz HSLV high speed @ 1.2V pulldown"
io8_166m_hslv_ft_fs_1v2  "IO8_FT 166MHz HSLV fast speed @ 1.2V"
io8_166m_hslv_ft_fs_pu_1v2  "IO8_FT 166MHz HSLV fast speed @ 1.2V pullup"
io8_166m_hslv_ft_fs_pd_1v2  "IO8_FT 166MHz HSLV fast speed @ 1.2V pulldown"
io8_166m_hslv_ft_ms_1v2  "IO8_FT 166MHz HSLV med speed @ 1.2V"
io8_166m_hslv_ft_ms_pu_1v2  "IO8_FT 166MHz HSLV med speed @ 1.2V pullup"
io8_166m_hslv_ft_ms_pd_1v2  "IO8_FT 166MHz HSLV med speed @ 1.2V pulldown"
io8_166m_hslv_ft_ls_1v2  "IO8_FT 166MHz HSLV low speed @ 1.2V"
io8_166m_hslv_ft_ls_pu_1v2  "IO8_FT 166MHz HSLV low speed @ 1.2V pullup"
io8_166m_hslv_ft_ls_pd_1v2  "IO8_FT 166MHz HSLV low speed @ 1.2V pulldown"
io8_166m_hslv_ft_hs_1v8  "IO8_FT 166MHz HSLV high speed @ 1.8V"
io8_166m_hslv_ft_hs_pu_1v8  "IO8_FT 166MHz HSLV high speed @ 1.8V pullup"
io8_166m_hslv_ft_hs_pd_1v8  "IO8_FT 166MHz HSLV high speed @ 1.8V pulldown"
io8_166m_hslv_ft_fs_1v8  "IO8_FT 166MHz HSLV fast speed @ 1.8V"
io8_166m_hslv_ft_fs_pu_1v8  "IO8_FT 166MHz HSLV fast speed @ 1.8V pullup"
io8_166m_hslv_ft_fs_pd_1v8  "IO8_FT 166MHz HSLV fast speed @ 1.8V pulldown"
io8_166m_hslv_ft_ms_1v8  "IO8_FT 166MHz HSLV med speed @ 1.8V"
io8_166m_hslv_ft_ms_pu_1v8  "IO8_FT 166MHz HSLV med speed @ 1.8V pullup"
io8_166m_hslv_ft_ms_pd_1v8  "IO8_FT 166MHz HSLV med speed @ 1.8V pulldown"
io8_166m_hslv_ft_ls_1v8  "IO8_FT 166MHz HSLV low speed @ 1.8V"
io8_166m_hslv_ft_ls_pu_1v8  "IO8_FT 166MHz HSLV low speed @ 1.8V pullup"
io8_166m_hslv_ft_ls_pd_1v8  "IO8_FT 166MHz HSLV low speed @ 1.8V pulldown"
io8_166m_hslv_ft_hs_2v5  "IO8_FT 166MHz HSLV high speed @ 2.5V"
io8_166m_hslv_ft_hs_pu_2v5  "IO8_FT 166MHz HSLV high speed @ 2.5V pullup"
io8_166m_hslv_ft_hs_pd_2v5  "IO8_FT 166MHz HSLV high speed @ 2.5V pulldown"
io8_166m_hslv_ft_fs_2v5  "IO8_FT 166MHz HSLV fast speed @ 2.5V"
io8_166m_hslv_ft_fs_pu_2v5  "IO8_FT 166MHz HSLV fast speed @ 2.5V pullup"
io8_166m_hslv_ft_fs_pd_2v5  "IO8_FT 166MHz HSLV fast speed @ 2.5V pulldown"
io8_166m_hslv_ft_ms_2v5  "IO8_FT 166MHz HSLV med speed @ 2.5V"
io8_166m_hslv_ft_ms_pu_2v5  "IO8_FT 166MHz HSLV med speed @ 2.5V pullup"
io8_166m_hslv_ft_ms_pd_2v5  "IO8_FT 166MHz HSLV med speed @ 2.5V pulldown"
io8_166m_hslv_ft_ls_2v5  "IO8_FT 166MHz HSLV low speed @ 2.5V"
io8_166m_hslv_ft_ls_pu_2v5  "IO8_FT 166MHz HSLV low speed @ 2.5V pullup"
io8_166m_hslv_ft_ls_pd_2v5  "IO8_FT 166MHz HSLV low speed @ 2.5V pulldown"
[Model Selector] io8_spi_hslv_ft
io8_spi_ft_hs_1v2  "IO8_FT SPI high speed @ 1.2V"
io8_spi_ft_hs_pu_1v2  "IO8_FT SPI high speed @ 1.2V pullup"
io8_spi_ft_hs_pd_1v2  "IO8_FT SPI high speed @ 1.2V pulldown"
io8_spi_ft_fs_1v2  "IO8_FT SPI fast speed @ 1.2V"
io8_spi_ft_fs_pu_1v2  "IO8_FT SPI fast speed @ 1.2V pullup"
io8_spi_ft_fs_pd_1v2  "IO8_FT SPI fast speed @ 1.2V pulldown"
io8_spi_ft_ms_1v2  "IO8_FT SPI med speed @ 1.2V"
io8_spi_ft_ms_pu_1v2  "IO8_FT SPI med speed @ 1.2V pullup"
io8_spi_ft_ms_pd_1v2  "IO8_FT SPI med speed @ 1.2V pulldown"
io8_spi_ft_ls_1v2  "IO8_FT SPI low speed @ 1.2V"
io8_spi_ft_ls_pu_1v2  "IO8_FT SPI low speed @ 1.2V pullup"
io8_spi_ft_ls_pd_1v2  "IO8_FT SPI low speed @ 1.2V pulldown"
io8_spi_ft_hs_1v8  "IO8_FT SPI high speed @ 1.8V"
io8_spi_ft_hs_pu_1v8  "IO8_FT SPI high speed @ 1.8V pullup"
io8_spi_ft_hs_pd_1v8  "IO8_FT SPI high speed @ 1.8V pulldown"
io8_spi_ft_fs_1v8  "IO8_FT SPI fast speed @ 1.8V"
io8_spi_ft_fs_pu_1v8  "IO8_FT SPI fast speed @ 1.8V pullup"
io8_spi_ft_fs_pd_1v8  "IO8_FT SPI fast speed @ 1.8V pulldown"
io8_spi_ft_ms_1v8  "IO8_FT SPI med speed @ 1.8V"
io8_spi_ft_ms_pu_1v8  "IO8_FT SPI med speed @ 1.8V pullup"
io8_spi_ft_ms_pd_1v8  "IO8_FT SPI med speed @ 1.8V pulldown"
io8_spi_ft_ls_1v8  "IO8_FT SPI low speed @ 1.8V"
io8_spi_ft_ls_pu_1v8  "IO8_FT SPI low speed @ 1.8V pullup"
io8_spi_ft_ls_pd_1v8  "IO8_FT SPI low speed @ 1.8V pulldown"
io8_spi_ft_hs_3v3  "IO8_FT SPI high speed @ 3.3V"
io8_spi_ft_hs_pu_3v3  "IO8_FT SPI high speed @ 3.3V pullup"
io8_spi_ft_hs_pd_3v3  "IO8_FT SPI high speed @ 3.3V pulldown"
io8_spi_ft_fs_3v3  "IO8_FT SPI fast speed @ 3.3V"
io8_spi_ft_fs_pu_3v3  "IO8_FT SPI fast speed @ 3.3V pullup"
io8_spi_ft_fs_pd_3v3  "IO8_FT SPI fast speed @ 3.3V pulldown"
io8_spi_ft_ms_3v3  "IO8_FT SPI med speed @ 3.3V"
io8_spi_ft_ms_pu_3v3  "IO8_FT SPI med speed @ 1.8V pullup"
io8_spi_ft_ms_pd_3v3  "IO8_FT SPI med speed @ 3.3V pulldown"
io8_spi_ft_ls_3v3  "IO8_FT SPI low speed @ 3.3V"
io8_spi_ft_ls_pu_3v3  "IO8_FT SPI low speed @ 3.3V pullup"
io8_spi_ft_ls_pd_3v3  "IO8_FT SPI low speed @ 3.3V pulldown"
io8_spi_hslv_ft_hs_1v2  "IO8_FT SPI HSLV high speed @ 1.2V"
io8_spi_hslv_ft_hs_pu_1v2  "IO8_FT SPI HSLV high speed @ 1.2V pullup"
io8_spi_hslv_ft_hs_pd_1v2  "IO8_FT SPI HSLV high speed @ 1.2V pulldown"
io8_spi_hslv_ft_fs_1v2  "IO8_FT SPI HSLV fast speed @ 1.2V"
io8_spi_hslv_ft_fs_pu_1v2  "IO8_FT SPI HSLV fast speed @ 1.2V pullup"
io8_spi_hslv_ft_fs_pd_1v2  "IO8_FT SPI HSLV fast speed @ 1.2V pulldown"
io8_spi_hslv_ft_ms_1v2  "IO8_FT SPI HSLV med speed @ 1.2V"
io8_spi_hslv_ft_ms_pu_1v2  "IO8_FT SPI HSLV med speed @ 1.2V pullup"
io8_spi_hslv_ft_ms_pd_1v2  "IO8_FT SPI HSLV med speed @ 1.2V pulldown"
io8_spi_hslv_ft_ls_1v2  "IO8_FT SPI HSLV low speed @ 1.2V"
io8_spi_hslv_ft_ls_pu_1v2  "IO8_FT SPI HSLV low speed @ 1.2V pullup"
io8_spi_hslv_ft_ls_pd_1v2  "IO8_FT SPI HSLV low speed @ 1.2V pulldown"
io8_spi_hslv_ft_hs_1v8  "IO8_FT SPI HSLV high speed @ 1.8V"
io8_spi_hslv_ft_hs_pu_1v8  "IO8_FT SPI HSLV high speed @ 1.8V pullup"
io8_spi_hslv_ft_hs_pd_1v8  "IO8_FT SPI HSLV high speed @ 1.8V pulldown"
io8_spi_hslv_ft_fs_1v8  "IO8_FT SPI HSLV fast speed @ 1.8V"
io8_spi_hslv_ft_fs_pu_1v8  "IO8_FT SPI HSLV fast speed @ 1.8V pullup"
io8_spi_hslv_ft_fs_pd_1v8  "IO8_FT SPI HSLV fast speed @ 1.8V pulldown"
io8_spi_hslv_ft_ms_1v8  "IO8_FT SPI HSLV med speed @ 1.8V"
io8_spi_hslv_ft_ms_pu_1v8  "IO8_FT SPI HSLV med speed @ 1.8V pullup"
io8_spi_hslv_ft_ms_pd_1v8  "IO8_FT SPI HSLV med speed @ 1.8V pulldown"
io8_spi_hslv_ft_ls_1v8  "IO8_FT SPI HSLV low speed @ 1.8V"
io8_spi_hslv_ft_ls_pu_1v8  "IO8_FT SPI HSLV low speed @ 1.8V pullup"
io8_spi_hslv_ft_ls_pd_1v8  "IO8_FT SPI HSLV low speed @ 1.8V pulldown"
io8_spi_hslv_ft_hs_2v5  "IO8_FT SPI HSLV high speed @ 2.5V"
io8_spi_hslv_ft_hs_pu_2v5  "IO8_FT SPI HSLV high speed @ 2.5V pullup"
io8_spi_hslv_ft_hs_pd_2v5  "IO8_FT SPI HSLV high speed @ 2.5V pulldown"
io8_spi_hslv_ft_fs_2v5  "IO8_FT SPI HSLV fast speed @ 2.5V"
io8_spi_hslv_ft_fs_pu_2v5  "IO8_FT SPI HSLV fast speed @ 2.5V pullup"
io8_spi_hslv_ft_fs_pd_2v5  "IO8_FT SPI HSLV fast speed @ 2.5V pulldown"
io8_spi_hslv_ft_ms_2v5  "IO8_FT SPI HSLV med speed @ 2.5V"
io8_spi_hslv_ft_ms_pu_2v5  "IO8_FT SPI HSLV med speed @ 2.5V pullup"
io8_spi_hslv_ft_ms_pd_2v5  "IO8_FT SPI HSLV med speed @ 2.5V pulldown"
io8_spi_hslv_ft_ls_2v5  "IO8_FT SPI HSLV low speed @ 2.5V"
io8_spi_hslv_ft_ls_pu_2v5  "IO8_FT SPI HSLV low speed @ 2.5V pullup"
io8_spi_hslv_ft_ls_pd_2v5  "IO8_FT SPI HSLV low speed @ 2.5V pulldown"
[Model Selector] io8_spi_ft
io8_spi_ft_hs_1v2  "IO8_FT SPI high speed @ 1.2V"
io8_spi_ft_hs_pu_1v2  "IO8_FT SPI high speed @ 1.2V pullup"
io8_spi_ft_hs_pd_1v2  "IO8_FT SPI high speed @ 1.2V pulldown"
io8_spi_ft_fs_1v2  "IO8_FT SPI fast speed @ 1.2V"
io8_spi_ft_fs_pu_1v2  "IO8_FT SPI fast speed @ 1.2V pullup"
io8_spi_ft_fs_pd_1v2  "IO8_FT SPI fast speed @ 1.2V pulldown"
io8_spi_ft_ms_1v2  "IO8_FT SPI med speed @ 1.2V"
io8_spi_ft_ms_pu_1v2  "IO8_FT SPI med speed @ 1.2V pullup"
io8_spi_ft_ms_pd_1v2  "IO8_FT SPI med speed @ 1.2V pulldown"
io8_spi_ft_ls_1v2  "IO8_FT SPI low speed @ 1.2V"
io8_spi_ft_ls_pu_1v2  "IO8_FT SPI low speed @ 1.2V pullup"
io8_spi_ft_ls_pd_1v2  "IO8_FT SPI low speed @ 1.2V pulldown"
io8_spi_ft_hs_1v8  "IO8_FT SPI high speed @ 1.8V"
io8_spi_ft_hs_pu_1v8  "IO8_FT SPI high speed @ 1.8V pullup"
io8_spi_ft_hs_pd_1v8  "IO8_FT SPI high speed @ 1.8V pulldown"
io8_spi_ft_fs_1v8  "IO8_FT SPI fast speed @ 1.8V"
io8_spi_ft_fs_pu_1v8  "IO8_FT SPI fast speed @ 1.8V pullup"
io8_spi_ft_fs_pd_1v8  "IO8_FT SPI fast speed @ 1.8V pulldown"
io8_spi_ft_ms_1v8  "IO8_FT SPI med speed @ 1.8V"
io8_spi_ft_ms_pu_1v8  "IO8_FT SPI med speed @ 1.8V pullup"
io8_spi_ft_ms_pd_1v8  "IO8_FT SPI med speed @ 1.8V pulldown"
io8_spi_ft_ls_1v8  "IO8_FT SPI low speed @ 1.8V"
io8_spi_ft_ls_pu_1v8  "IO8_FT SPI low speed @ 1.8V pullup"
io8_spi_ft_ls_pd_1v8  "IO8_FT SPI low speed @ 1.8V pulldown"
io8_spi_ft_hs_3v3  "IO8_FT SPI high speed @ 3.3V"
io8_spi_ft_hs_pu_3v3  "IO8_FT SPI high speed @ 3.3V pullup"
io8_spi_ft_hs_pd_3v3  "IO8_FT SPI high speed @ 3.3V pulldown"
io8_spi_ft_fs_3v3  "IO8_FT SPI fast speed @ 3.3V"
io8_spi_ft_fs_pu_3v3  "IO8_FT SPI fast speed @ 3.3V pullup"
io8_spi_ft_fs_pd_3v3  "IO8_FT SPI fast speed @ 3.3V pulldown"
io8_spi_ft_ms_3v3  "IO8_FT SPI med speed @ 3.3V"
io8_spi_ft_ms_pu_3v3  "IO8_FT SPI med speed @ 1.8V pullup"
io8_spi_ft_ms_pd_3v3  "IO8_FT SPI med speed @ 3.3V pulldown"
io8_spi_ft_ls_3v3  "IO8_FT SPI low speed @ 3.3V"
io8_spi_ft_ls_pu_3v3  "IO8_FT SPI low speed @ 3.3V pullup"
io8_spi_ft_ls_pd_3v3  "IO8_FT SPI low speed @ 3.3V pulldown"
io8_spi_hslv_ft_hs_1v2  "IO8_FT SPI HSLV high speed @ 1.2V"
io8_spi_hslv_ft_hs_pu_1v2  "IO8_FT SPI HSLV high speed @ 1.2V pullup"
io8_spi_hslv_ft_hs_pd_1v2  "IO8_FT SPI HSLV high speed @ 1.2V pulldown"
io8_spi_hslv_ft_fs_1v2  "IO8_FT SPI HSLV fast speed @ 1.2V"
io8_spi_hslv_ft_fs_pu_1v2  "IO8_FT SPI HSLV fast speed @ 1.2V pullup"
io8_spi_hslv_ft_fs_pd_1v2  "IO8_FT SPI HSLV fast speed @ 1.2V pulldown"
io8_spi_hslv_ft_ms_1v2  "IO8_FT SPI HSLV med speed @ 1.2V"
io8_spi_hslv_ft_ms_pu_1v2  "IO8_FT SPI HSLV med speed @ 1.2V pullup"
io8_spi_hslv_ft_ms_pd_1v2  "IO8_FT SPI HSLV med speed @ 1.2V pulldown"
io8_spi_hslv_ft_ls_1v2  "IO8_FT SPI HSLV low speed @ 1.2V"
io8_spi_hslv_ft_ls_pu_1v2  "IO8_FT SPI HSLV low speed @ 1.2V pullup"
io8_spi_hslv_ft_ls_pd_1v2  "IO8_FT SPI HSLV low speed @ 1.2V pulldown"
io8_spi_hslv_ft_hs_1v8  "IO8_FT SPI HSLV high speed @ 1.8V"
io8_spi_hslv_ft_hs_pu_1v8  "IO8_FT SPI HSLV high speed @ 1.8V pullup"
io8_spi_hslv_ft_hs_pd_1v8  "IO8_FT SPI HSLV high speed @ 1.8V pulldown"
io8_spi_hslv_ft_fs_1v8  "IO8_FT SPI HSLV fast speed @ 1.8V"
io8_spi_hslv_ft_fs_pu_1v8  "IO8_FT SPI HSLV fast speed @ 1.8V pullup"
io8_spi_hslv_ft_fs_pd_1v8  "IO8_FT SPI HSLV fast speed @ 1.8V pulldown"
io8_spi_hslv_ft_ms_1v8  "IO8_FT SPI HSLV med speed @ 1.8V"
io8_spi_hslv_ft_ms_pu_1v8  "IO8_FT SPI HSLV med speed @ 1.8V pullup"
io8_spi_hslv_ft_ms_pd_1v8  "IO8_FT SPI HSLV med speed @ 1.8V pulldown"
io8_spi_hslv_ft_ls_1v8  "IO8_FT SPI HSLV low speed @ 1.8V"
io8_spi_hslv_ft_ls_pu_1v8  "IO8_FT SPI HSLV low speed @ 1.8V pullup"
io8_spi_hslv_ft_ls_pd_1v8  "IO8_FT SPI HSLV low speed @ 1.8V pulldown"
io8_spi_hslv_ft_hs_2v5  "IO8_FT SPI HSLV high speed @ 2.5V"
io8_spi_hslv_ft_hs_pu_2v5  "IO8_FT SPI HSLV high speed @ 2.5V pullup"
io8_spi_hslv_ft_hs_pd_2v5  "IO8_FT SPI HSLV high speed @ 2.5V pulldown"
io8_spi_hslv_ft_fs_2v5  "IO8_FT SPI HSLV fast speed @ 2.5V"
io8_spi_hslv_ft_fs_pu_2v5  "IO8_FT SPI HSLV fast speed @ 2.5V pullup"
io8_spi_hslv_ft_fs_pd_2v5  "IO8_FT SPI HSLV fast speed @ 2.5V pulldown"
io8_spi_hslv_ft_ms_2v5  "IO8_FT SPI HSLV med speed @ 2.5V"
io8_spi_hslv_ft_ms_pu_2v5  "IO8_FT SPI HSLV med speed @ 2.5V pullup"
io8_spi_hslv_ft_ms_pd_2v5  "IO8_FT SPI HSLV med speed @ 2.5V pulldown"
io8_spi_hslv_ft_ls_2v5  "IO8_FT SPI HSLV low speed @ 2.5V"
io8_spi_hslv_ft_ls_pu_2v5  "IO8_FT SPI HSLV low speed @ 2.5V pullup"
io8_spi_hslv_ft_ls_pd_2v5  "IO8_FT SPI HSLV low speed @ 2.5V pulldown"
[Define Package Model]  481-ufbga-7x7-132-ldo-220909
[Manufacturer]  unknown
[OEM]  unknown
[Description]  unknown
[Number Of Pins]  122
[Pin Numbers]
| Pin Name Terminal   Net Name   Starting Node   Ending Node
G2 | NRST
H3 | OPAMP1_VINM
M2 | OPAMP2_VINM
J2 | PA0
G4 | PA1
K2 | PA2
L1 | PA3
L3 | PA4
M1 | PA5
L2 | PA6
K3 | PA7
D12 | PA8
D10 | PA9
D11 | PA10
C12 | PA11
B12 | PA12
C10 | PA13
C11 | PA14
A11 | PA15
M4 | PB0
L4 | PB1
K4 | PB2
C6 | PB3
B6 | PB4
D6 | PB5
A5 | PB6
D5 | PB7
C5 | PB8
A4 | PB9
K9 | PB10
L9 | PB11
L11 | PB12
K10 | PB13
K11 | PB14
K12 | PB15
H2 | PC0
G3 | PC1
F3 | PC2
F4 | PC3
M3 | PC4
J3 | PC5
F11 | PC6
E10 | PC7
E12 | PC8
E11 | PC9
B11 | PC10
A10 | PC11
B10 | PC12
C3 | PC13
C1 | PC14-OSC32_IN
D1 | PC15-OSC32_OUT
C9 | PD0
B9 | PD1
A9 | PD2
C8 | PD3
B8 | PD4
A8 | PD5
A7 | PD6
D7 | PD7
L12 | PD8
J10 | PD9
M12 | PD10
J11 | PD11
J12 | PD12
H11 | PD13
H10 | PD14
H12 | PD15
C4 | PE0
A3 | PE1
B3 | PE2
A2 | PE3
B2 | PE4
A1 | PE5
C2 | PE6
K7 | PE7
J6 | PE8
M7 | PE9
J7 | PE10
L7 | PE11
J8 | PE12
M8 | PE13
K8 | PE14
L8 | PE15
D2 | PF0
E2 | PF1
E1 | PF2
D3 | PF3
E3 | PF4
F2 | PF5
K5 | PF11
L5 | PF12
M5 | PF13
J5 | PF14
L6 | PF15
M6 | PG0
K6 | PG1
G10 | PG2
G11 | PG3
G9 | PG4
G12 | PG5
F9 | PG6
F10 | PG7
F12 | PG8
B7 | PG9
C7 | PG10
M11 | PG11
A6 | PG12
M10 | PG13
M9 | PG14
B4 | PG15
F1 | PH0-OSC_IN
G1 | PH1-OSC_OUT
B5 | PH3
L10 | VCAP
B1 | VBAT
D4 | VDD
K1 | VDDA
D8 | VDDIO2
A12 | VDDUSB
J1 | VREFP
E4 | VSS
H1 | VSSA_VREFM
|[Merged Pins]  D4
|D9  |  VDD
|F7  |  VDD
|G6  |  VDD
|J4  |  VDD
|J9  |  VDD
|[Merged Pins]  E4
|E9  |  VSS
|F6  |  VSS
|G7  |  VSS
|H4  |  VSS
|H9  |  VSS
[Model Data]
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[End Model Data]
[End Package Model]
| Models and submodels in the file (265): io8_100m_ft_hs_1v2 (I/O), io8_100m_ft_hs_pu_1v2 (I/O), io8_100m_ft_hs_pd_1v2 (I/O), io8_100m_ft_fs_1v2 (I/O), io8_100m_ft_fs_pu_1v2 (I/O), io8_100m_ft_fs_pd_1v2 (I/O), io8_100m_ft_ms_1v2 (I/O), io8_100m_ft_ms_pu_1v2 (I/O), io8_100m_ft_ms_pd_1v2 (I/O), io8_100m_ft_ls_1v2 (I/O), io8_100m_ft_ls_pu_1v2 (I/O), io8_100m_ft_ls_pd_1v2 (I/O), io8_100m_ft_hs_1v8 (I/O), io8_100m_ft_hs_pu_1v8 (I/O), io8_100m_ft_hs_pd_1v8 (I/O), io8_100m_ft_fs_1v8 (I/O), io8_100m_ft_fs_pu_1v8 (I/O), io8_100m_ft_fs_pd_1v8 (I/O), io8_100m_ft_ms_1v8 (I/O), io8_100m_ft_ms_pu_1v8 (I/O), io8_100m_ft_ms_pd_1v8 (I/O), io8_100m_ft_ls_1v8 (I/O), io8_100m_ft_ls_pu_1v8 (I/O), io8_100m_ft_ls_pd_1v8 (I/O), io8_100m_ft_hs_3v3 (I/O), io8_100m_ft_hs_pu_3v3 (I/O), io8_100m_ft_hs_pd_3v3 (I/O), io8_100m_ft_fs_3v3 (I/O), io8_100m_ft_fs_pu_3v3 (I/O), io8_100m_ft_fs_pd_3v3 (I/O), io8_100m_ft_ms_3v3 (I/O), io8_100m_ft_ms_pu_3v3 (I/O), io8_100m_ft_ms_pd_3v3 (I/O), io8_100m_ft_ls_3v3 (I/O), io8_100m_ft_ls_pu_3v3 (I/O), io8_100m_ft_ls_pd_3v3 (I/O), io8_100m_hslv_ft_hs_1v2 (I/O), io8_100m_hslv_ft_hs_pu_1v2 (I/O), io8_100m_hslv_ft_hs_pd_1v2 (I/O), io8_100m_hslv_ft_fs_1v2 (I/O), io8_100m_hslv_ft_fs_pu_1v2 (I/O), io8_100m_hslv_ft_fs_pd_1v2 (I/O), io8_100m_hslv_ft_ms_1v2 (I/O), io8_100m_hslv_ft_ms_pu_1v2 (I/O), io8_100m_hslv_ft_ms_pd_1v2 (I/O), io8_100m_hslv_ft_ls_1v2 (I/O), io8_100m_hslv_ft_ls_pu_1v2 (I/O), io8_100m_hslv_ft_ls_pd_1v2 (I/O), io8_100m_hslv_ft_hs_1v8 (I/O), io8_100m_hslv_ft_hs_pu_1v8 (I/O), io8_100m_hslv_ft_hs_pd_1v8 (I/O), io8_100m_hslv_ft_fs_1v8 (I/O), io8_100m_hslv_ft_fs_pu_1v8 (I/O), io8_100m_hslv_ft_fs_pd_1v8 (I/O), io8_100m_hslv_ft_ms_1v8 (I/O), io8_100m_hslv_ft_ms_pu_1v8 (I/O), io8_100m_hslv_ft_ms_pd_1v8 (I/O), io8_100m_hslv_ft_ls_1v8 (I/O), io8_100m_hslv_ft_ls_pu_1v8 (I/O), io8_100m_hslv_ft_ls_pd_1v8 (I/O), io8_100m_hslv_ft_hs_2v5 (I/O), io8_100m_hslv_ft_hs_pu_2v5 (I/O), io8_100m_hslv_ft_hs_pd_2v5 (I/O), io8_100m_hslv_ft_fs_2v5 (I/O), io8_100m_hslv_ft_fs_pu_2v5 (I/O), io8_100m_hslv_ft_fs_pd_2v5 (I/O), io8_100m_hslv_ft_ms_2v5 (I/O), io8_100m_hslv_ft_ms_pu_2v5 (I/O), io8_100m_hslv_ft_ms_pd_2v5 (I/O), io8_100m_hslv_ft_ls_2v5 (I/O), io8_100m_hslv_ft_ls_pu_2v5 (I/O), io8_100m_hslv_ft_ls_pd_2v5 (I/O), io8_100m_i2c_ft_1v2 (I/O_open_drain), io8_100m_i2c_ft_pu_1v2 (I/O_open_drain), io8_100m_i2c_ft_pd_1v2 (I/O_open_drain), io8_100m_i2c_ft_1v8 (I/O_open_drain), io8_100m_i2c_ft_pu_1v8 (I/O_open_drain), io8_100m_i2c_ft_pd_1v8 (I/O_open_drain), io8_100m_i2c_ft_3v3 (I/O_open_drain), io8_100m_i2c_ft_pu_3v3 (I/O_open_drain)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
